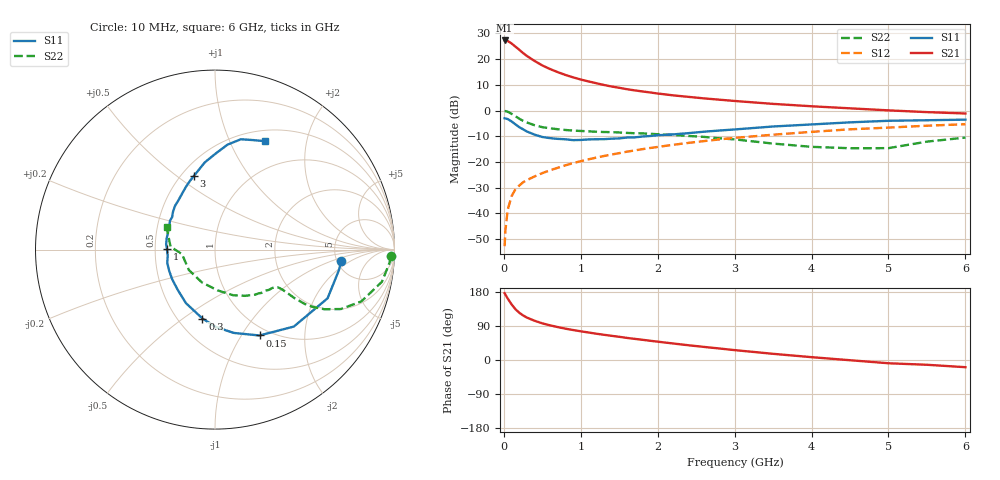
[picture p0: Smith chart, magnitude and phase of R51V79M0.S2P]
! SIEMENS Small Signal Semiconductors
! BFR183
! Si NPN RF Bipolar Junction Transistor in SOT23
! VCE = 1.75 V  IC = 9 mA
! Common Emitter S-Parameters:  May  1996
# GHz  S  MA  R  50
!  f  S11  S21  S12  S22
! GHz  MAG  ANG  MAG  ANG  MAG  ANG  MAG  ANG
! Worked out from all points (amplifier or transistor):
!   36 points, 10 MHz to 6 GHz, reference 50 ohm
!   highest |S21| = 27.3 dB at 10 MHz (marker M1)
!   |S21| within 3 dB of that: start of sweep to 175.4 MHz
!   unconditionally stable (mu >= 1): 789.1 MHz to 2.538 GHz
!   at 250 MHz: K = 0.60, MSG = 25.1 dB, |S12| = -27.9 dB
!   at 1.4 GHz: K = 1.06, MAG = 11.7 dB, |S12| = -17.1 dB
!   at 6 GHz: K = 0.90, MSG = 2.1 dB, |S12| = -5.3 dB
!   S11 on the Smith chart (normalised r, x): 10 MHz: 5.46, -1.37; 150 MHz: 0.89, -1.20; 300 MHz: 0.66, -0.59; 1 GHz: 0.58, +0.00; 3 GHz: 0.58, +0.58; 6 GHz: 0.63, +1.36
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0.01  0.7067 -5.1  23.05 176.4  0.0023 85.4  0.9814 -2.2
0.02  0.7001 -9.3  22.87 172.6  0.0046 83.1  0.9748 -4.4
0.05  0.6834 -23.4  22.5 162.3  0.0117 79.4  0.9472 -10.9
0.1  0.6139 -44.3  20.19 147.0  0.0215 71.9  0.865 -19.5
0.15  0.539 -62.6  17.53 134.2  0.0293 65.5  0.7751 -25.3
0.2  0.4759 -77.3  15.22 124.8  0.0347 62.6  0.6939 -28.6
0.25  0.4313 -89.3  13.13 117.6  0.0402 61.3  0.6308 -30.4
0.3  0.3905 -100.3  11.51 111.9  0.0443 60.7  0.5853 -31.2
0.4  0.3394 -118.5  9.194 103.5  0.0523 60.8  0.517 -31.4
0.5  0.3053 -133.0  7.531 96.7  0.0606 61.9  0.4745 -31.0
0.6  0.2903 -145.3  6.415 91.5  0.0688 62.7  0.4506 -30.8
0.7  0.281 -155.7  5.584 86.9  0.0769 63.2  0.433 -30.7
0.8  0.276 -164.5  4.923 82.7  0.0859 63.2  0.4185 -30.8
1  0.2678 179.5  4.008 75.7  0.1033 64.2  0.4002 -31.5
1.1  0.2739 173.6  3.682 72.6  0.1123 64.0  0.3938 -32.6
1.6  0.2981 147.3  2.597 58.3  0.1582 61.6  0.3669 -38.3
2.2  0.3431 126.2  1.973 43.6  0.2154 56.9  0.3356 -48.5
3  0.4284 105.7  1.534 26.1  0.2935 48.3  0.2745 -68.1
3.5  0.4892 96.7  1.346 16.3  0.3386 42.0  0.2276 -86.4
4.5  0.5888 83.2  1.103 -0.6  0.431 29.4  0.1847 -142.0
5.5  0.647 70.5  0.931 -12.6  0.5068 17.4  0.2482 176.2
6  0.6643 65.4  0.875 -19.0  0.5416 9.5  0.2977 155.1
